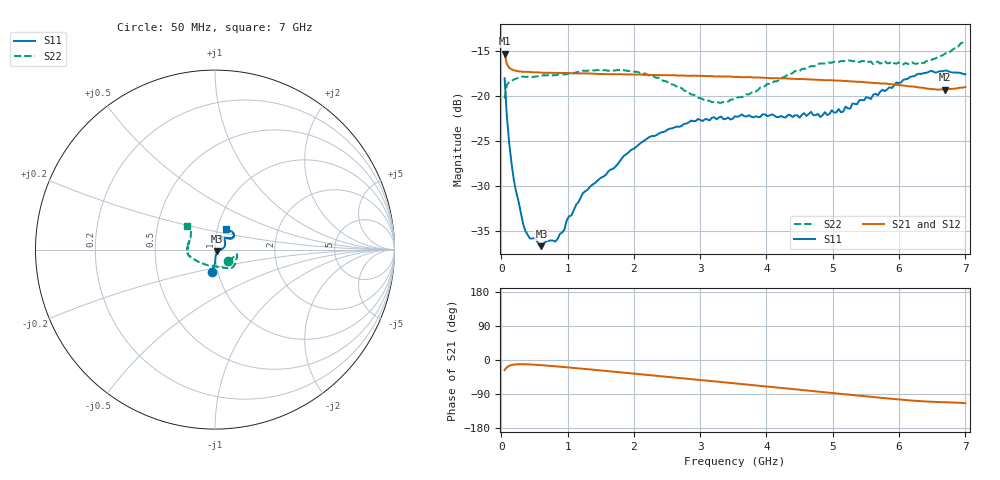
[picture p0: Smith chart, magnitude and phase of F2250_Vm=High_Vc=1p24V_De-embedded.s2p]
! Integrated Device Technology
! Corporate Headquarters
! 6024 Silver Creek Valley Road
! San Jose, CA 95138  USA
! Phone:  1-408-284-8200
! Toll Free:  1-800-223-1366
! Webpage:  http://www.idt.com/
! Timing and RF Division
! 515 Groton Road, Suite 102
! Westford, MA 01886-6024
! Device:  F2250
! Description: Voltage Variable RF Attenuator
! Frequency:  50.0 -  6000.00 MHz
! Package:  3x3 mm Thin QFN Plastic Package: 16 pin
! Ports:  2 RF, 3 DC
!  Pin  1  = GND
!  Pin  2  = NC
!  Pin  3  = RF1  = Port 1
!  Pin  4  = NC
!  Pin  5  = GND
!  Pin  6  = GND
!  Pin  7  = GND
!  Pin  8  = GND
!  Pin  9  = NC
!  Pin 10  = RF2  = Port 2
!  Pin 11  = NC
!  Pin 12  = GND
!  Pin 13  = GND
!  Pin 14  = VCNTRL
!  Pin 15  = VDD
!  Pin 16  = VMODE
! Vcntrl:  1.240 Volts
! Vmode:  +3.300 Volts
! Vdd:  +3.30  Volts
! Current:  1.332 mA
! Data:  The device was measured on a the F2250 evaluation board which has
!  individual transmission lines to the RF pins.  Data was collected
!  using a calibrated network analyzer.  The evaluation board was
!  de-embedded using a TRL calibration technique.
!  The reference plane is the edge of the package pin.
! Misc:  SN 10
!  Action Tracker AT0258
! Date Measured:  2014-11-26
! Date:  2015-10-15  MJV
! Note:
!  Integrated Device Technology supplies this data as a sample of measured
!  data at the package pin for this product.  Your particular data for this
!  product may vary.
!  Data was taken at 25 degrees C.
!  Integrated Device Technology reserves the right to change this data at anytime.
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# GHz S dB R 50
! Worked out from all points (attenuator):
!   201 points, 50 MHz to 7 GHz, reference 50 ohm
!   highest |S21| = -15.31 dB at 50 MHz (marker M1); lowest = -19.3 dB at 6.687 GHz (marker M2)
!   lowest |S11| = -36.7 dB at 606 MHz (marker M3), VSWR 1.03, Z = 51.2 - j0.833 ohm
!   |S11| at or under -10 dB: start of sweep to end of sweep
!   |S22| runs from -20.8 to -13.8 dB; largest |S21 - S12| = 0.00054
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0.05  -18.04 -97.7  -15.31 -26.6  -15.29 -26.5  -20.30 -40.0
0.08475  -22.36 -89.9  -16.48 -19.1  -16.47 -19.1  -18.76 -19.4
0.15425  -27.48 -85.9  -17.06 -13.2  -17.06 -13.2  -18.36 -12.4
0.189  -29.35 -82.0  -17.17 -12.1  -17.15 -12.1  -18.18 -12.1
0.328  -34.19 -62.0  -17.33 -11.1  -17.33 -11.1  -17.86 -12.9
0.43225  -35.85 -56.7  -17.35 -11.7  -17.36 -11.7  -17.89 -14.3
0.606  -36.71 -33.8  -17.43 -13.7  -17.41 -13.7  -17.77 -19.6
0.84925  -35.90 -19.4  -17.45 -17.1  -17.44 -17.1  -17.66 -26.5
1.2315  -30.80 -7.7  -17.50 -23.1  -17.49 -23.1  -17.21 -35.3
1.96125  -26.00 13.7  -17.62 -35.0  -17.64 -35.0  -17.26 -47.9
2.37825  -24.18 24.6  -17.69 -42.0  -17.70 -42.0  -17.98 -56.3
3.07325  -22.58 46.2  -17.79 -53.9  -17.80 -53.9  -20.53 -85.5
3.525  -22.27 60.1  -17.90 -61.7  -17.89 -61.7  -20.33 -117.0
4.7065  -22.15 66.7  -18.19 -82.2  -18.20 -82.1  -16.72 -165.3
5.15825  -21.74 49.7  -18.36 -90.0  -18.37 -90.0  -16.12 -174.5
5.193  -21.20 49.8  -18.36 -90.6  -18.37 -90.6  -16.17 -175.4
5.2625  -21.42 46.5  -18.38 -91.8  -18.40 -91.8  -16.07 -176.3
5.29725  -20.86 45.7  -18.41 -92.4  -18.41 -92.4  -16.17 -177.2
5.85325  -19.06 35.1  -18.69 -101.8  -18.70 -101.9  -16.38 169.1
6.3745  -17.47 37.4  -19.12 -109.3  -19.15 -109.3  -16.35 151.7
6.68725  -17.20 45.4  -19.32 -111.4  -19.31 -111.5  -15.34 141.8
7  -17.61 62.4  -19.02 -113.9  -19.02 -114.1  -13.85 140.1
